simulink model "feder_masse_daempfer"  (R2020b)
settings: Solver=VariableStepAuto  StartTime=0.0  StopTime=10.0  RelTol=1e-6
model workspace (MAT data in the model file):
  c = 100
  k = 0.8

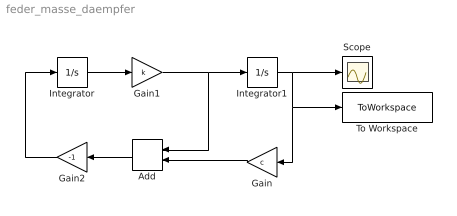
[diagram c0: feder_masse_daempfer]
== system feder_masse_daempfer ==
  Add : Sum
  Gain : Gain  Gain=c
  Gain1 : Gain  Gain=k
  Gain2 : Gain  Gain=-1
  Integrator : Integrator
  Integrator1 : Integrator  InitialCondition=0.1
  Scope : Scope
  To Workspace : ToWorkspace  VariableName=simout  SaveFormat=Timeseries  SampleTime=-1
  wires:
  Integrator1/1 -> Scope/1, To Workspace/1, Gain/1
  Integrator/1 -> Gain1/1
  Gain1/1 -> Integrator1/1, Add/1
  Gain/1 -> Add/2
  Add/1 -> Gain2/1
  Gain2/1 -> Integrator/1
